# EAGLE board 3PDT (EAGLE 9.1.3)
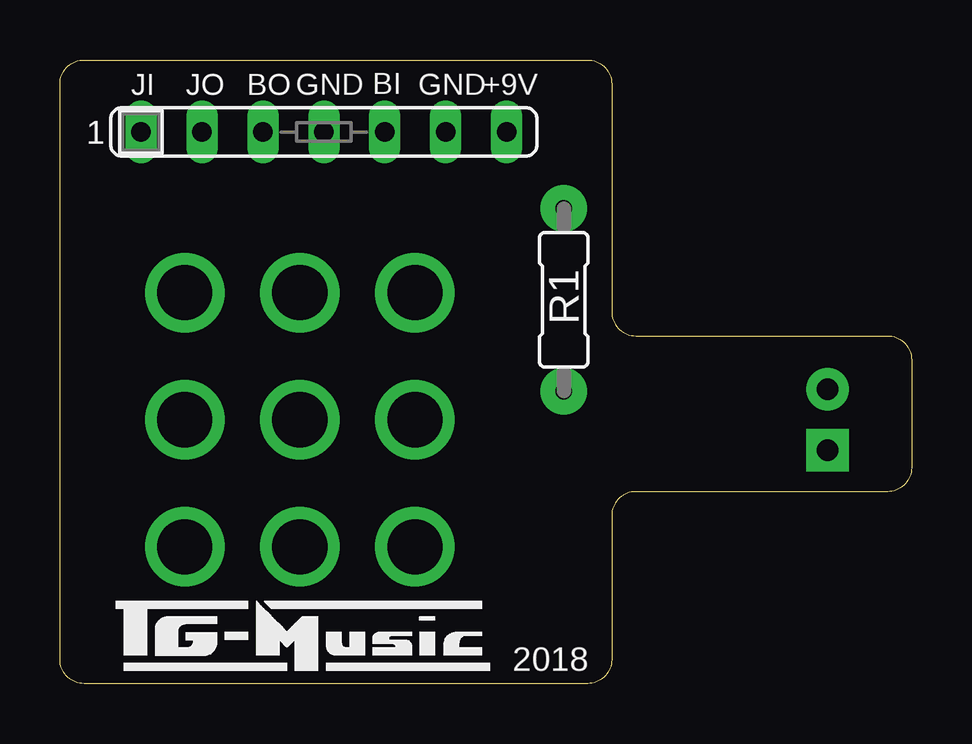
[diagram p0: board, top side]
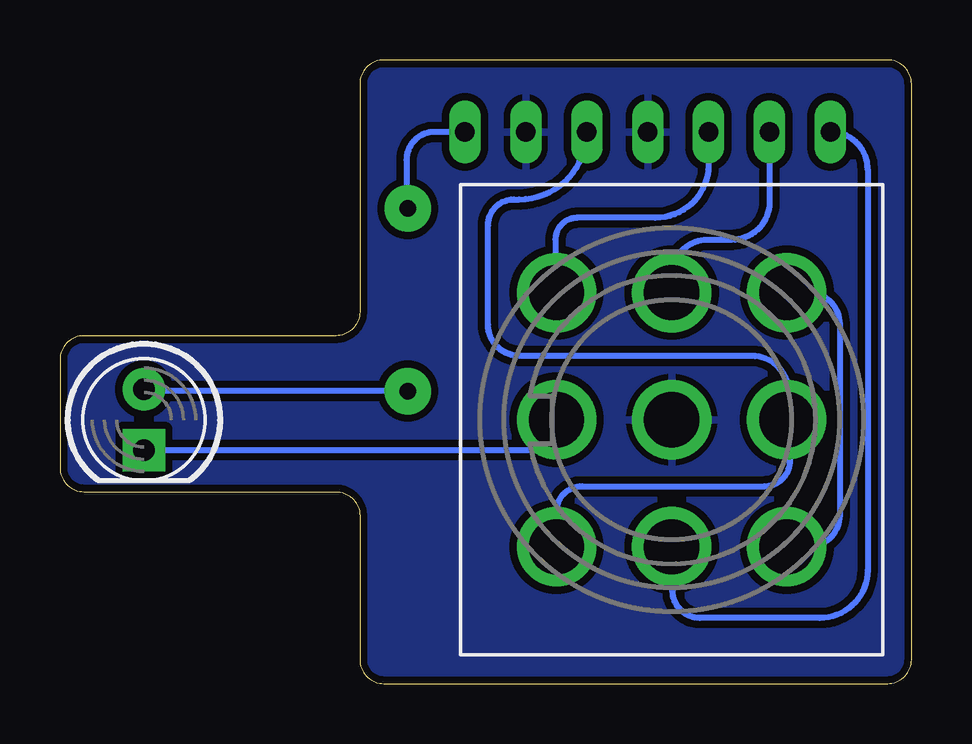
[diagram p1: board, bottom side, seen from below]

Size 35.5 x 26 mm. Coordinates in mm from the lower left corner, seen from the top.
Outline: 0,1 0,25 arc-90 1,26 22,26 arc-90 23,25 23,15.5 arc90 24,14.5 34.5,14.5 arc-90 35.5,13.5 35.5,9 arc-90 34.5,8 24,8 arc90 23,7 23,1 arc-90 22,0 1,0 arc-90 0,1
Copper layers (1*16): Top 0.035mm / dielectric 1.5mm / Bottom 0.035mm
Design rules "ITEADstudio": minimum track width 10mil, minimum drill 12mil, track to track 12mil, track to pad 12mil, pad to pad 12mil, via to via 12mil, smd to smd 0mil, copper to edge 12mil, drill to drill 12mil, minimum pad ring 10mil, minimum via ring 6mil, stop-mask expansion 4mil, vias tented up to drill 100mil, thermal gap 10mil

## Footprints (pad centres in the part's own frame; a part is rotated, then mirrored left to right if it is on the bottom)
3PDT = drill 2.3 pad 3.1: 1 -5.3,4.8; 2 0,4.8; 3 5.3,4.8; 4 -5.3,0; 5 0,0; 6 5.3,0; 7 -5.3,-4.8; 8 0,-4.8; 9 5.3,-4.8
SIL7 = drill 0.813 long: 1 -7.62,0; 2 -5.08,0; 3 -2.54,0; 4 0,0; 5 2.54,0; 6 5.08,0; 7 7.62,0
LED5MM = drill 0.9 pad 1.778: A -1.27,0 | drill 0.9 pad 1.778 square: K 1.27,0
R0207/3 = drill 0.7 pad 1.93: 1 -3.81,0; 2 3.81,0

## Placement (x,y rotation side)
E$1  [3PDT]  10,11 270 bottom
E$2  [SIL7]  11,23 0 top
E$3  [LED5MM]  32,11 270 bottom
R1  [R0207/3]  21,16 90 top

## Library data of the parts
E$1 = switch
E$2 = resistor-sil
E$3 = Diodit
R1 = Vastukset

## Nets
GND: E$1.5 E$2.4 E$2.6
S$1: E$1.1 E$1.3
S$2: E$1.4 E$2.2
S$3: E$1.7 E$2.3
S$4: E$1.2 E$1.9 E$2.5
S$5: E$1.6 E$2.1
S$7: E$1.8 E$3.K
S$8: E$2.7 R1.2
S$9: E$3.A R1.1

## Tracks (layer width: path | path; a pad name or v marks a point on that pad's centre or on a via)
GND
  pour Bottom: 0,1 0,25 arc-90 1,26 22,26 arc-90 23,25 23,15.5 arc90 24,14.5 34.5,14.5 arc-90 35.5,13.5 35.5,9 arc-90 34.5,8 24,8 arc90 23,7 23,1 arc-90 22,0 1,0 arc-90
S$1
  Bottom 0.254: E$1.1 4.3,16.3 arc90 3,15 3,7.01 arc90 4.32,5.68 5.18,5.68 arc90 E$1.3
S$2
  Bottom 0.254: E$2.2 5.92,20.08 arc90 7.5,18.5 8.5,18.5 arc-90 10,17 E$1.4
S$3
  Bottom 0.254: E$2.3 8.46,21.64 arc90 10.68,19.42 13.94,19.42 arc-90 14.85,18.51 14.85,16.34 arc-90 E$1.7
S$4
  Bottom 0.254: E$1.9 14.8,7.17 arc90 13.74,8.23 6.13,8.23 arc-90 5.06,9.29 5.06,10.93 arc-90 5.13,11 E$1.2 5.11,11.1 5.11,12.11 arc-90 6.66,13.66 16.35,13.66 arc90 17.65,14.96 17.65,19.11 arc90 16.58,20.19 16.35,20.19 arc-90 E$2.5
S$5
  Bottom 0.254: E$1.6 arc90 9.96,5.66 9.96,3.87 arc-90 8.82,2.74 3.83,2.74 arc-90 1.83,4.74 1.83,21.45 arc-90 E$2.1
S$7
  Bottom 0.254: E$3.K 16.07,9.73 arc-90 E$1.8
S$8
  Bottom 0.254: E$2.7 19.88,23 arc-90 21.05,21.83 21.05,19.86 arc-90 R1.2
S$9
  Bottom 0.254: R1.1 31.92,12.19 arc90 E$3.A

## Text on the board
tNames: JI | JO | BO | GND | BI | GND | +9V | 2018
